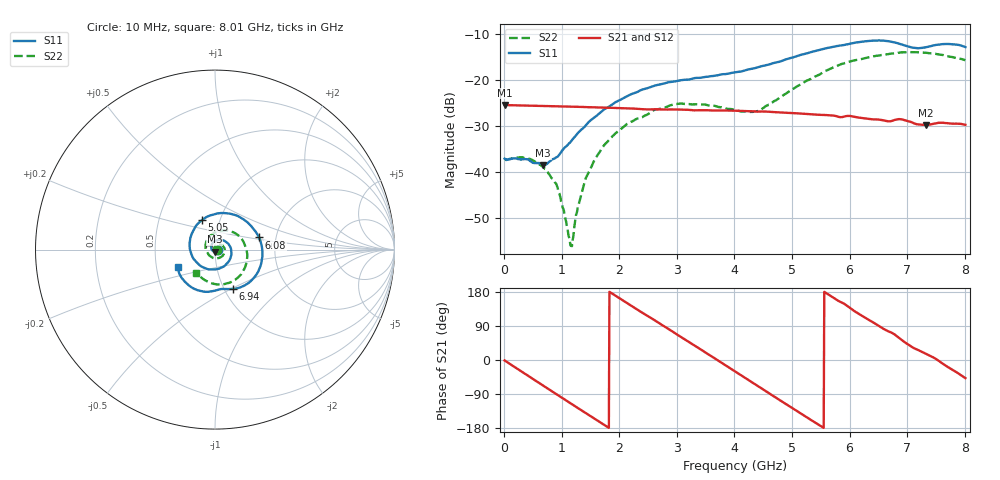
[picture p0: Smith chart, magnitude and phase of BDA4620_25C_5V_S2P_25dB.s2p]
!Agilent Technologies,E5071B,MY42404982,A.09.10
!Date: Wed May 06 09:03:50 2026
!Data & Calibration Information:
!Freq	S11:SOLT2(ON)	S21:SOLT2(ON)	S12:SOLT2(ON)	S22:SOLT2(ON)
# Hz S RI R 50
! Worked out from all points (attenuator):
!   801 points, 10 MHz to 8.01 GHz, reference 50 ohm
!   highest |S21| = -25.39 dB at 10 MHz (marker M1); lowest = -29.7 dB at 7.33 GHz (marker M2)
!   lowest |S11| = -38.5 dB at 680 MHz (marker M3), VSWR 1.02, Z = 49.8 - j1.16 ohm
!   |S11| at or under -10 dB: start of sweep to end of sweep
!   |S22| runs from -56.1 to -13.9 dB; largest |S21 - S12| = 0.00026
!   S11 on the Smith chart (normalised r, x): 10 MHz: 1.03, -0.00; 5.05 GHz: 0.82, +0.28; 6.08 GHz: 1.63, +0.24; 6.94 GHz: 1.09, -0.51; 8.01 GHz: 0.64, -0.13
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1e7  0.014 -0.000933  0.0538 -0.00111  0.0538 -0.00113  0.0135 -0.000458
4.2e8  0.00827 -0.0109  0.0394 -0.0354  0.0395 -0.0355  0.0132 -0.00462
6.8e8  -0.00218 -0.0117  0.02 -0.0486  0.02 -0.0487  0.00917 -0.00659
9.3e8  -0.0137 -0.00542  -0.00201 -0.0521  -0.00205 -0.0522  0.00349 -0.00588
1.16e9  -0.0202 0.00753  -0.0216 -0.0468  -0.0217 -0.0469  -0.00137 -0.000793
1.19e9  -0.0207 0.00964  -0.024 -0.0456  -0.024 -0.0457  -0.00181 0.000112
1.35e9  -0.0204 0.0211  -0.0352 -0.0372  -0.0352 -0.0373  -0.00332 0.00496
1.53e9  -0.0146 0.0348  -0.0444 -0.0247  -0.0444 -0.0248  -0.00307 0.0115
1.77e9  0.00199 0.0493  -0.05 -0.00514  -0.0501 -0.0051  0.00102 0.0207
2.14e9  0.0413 0.053  -0.0427 0.0248  -0.0428 0.0249  0.0169 0.0291
2.68e9  0.0891 0.00418  -0.00706 0.0476  -0.00703 0.0477  0.0445 0.0192
3.08e9  0.0812 -0.0587  0.024 0.0415  0.0242 0.0414  0.0551 -0.00764
4.01e9  -0.0835 -0.0886  0.0403 -0.0233  0.0404 -0.0234  -0.0108 -0.0465
4.43e9  -0.1396 0.00125  0.0151 -0.043  0.0151 -0.0431  -0.0451 -0.0114
5.05e9  -0.0729 0.164  -0.0288 -0.033  -0.0289 -0.033  -0.0253 0.0787
5.35e9  0.0212 0.2024  -0.04 -0.0144  -0.0401 -0.0144  0.0232 0.1022
6.08e9  0.2451 0.0679  -0.0254 0.0309  -0.0255 0.031  0.1577 0.0456
6.68e9  0.1933 -0.1811  0.00909 0.0345  0.0092 0.0346  0.1698 -0.09
6.94e9  0.098 -0.2196  0.0244 0.0278  0.0245 0.0278  0.1371 -0.1468
7.33e9  0.00168 -0.2279  0.0314 0.00912  0.0314 0.00921  0.0462 -0.193
7.65e9  -0.1156 -0.2187  0.0334 -0.00775  0.0335 -0.00776  -0.0329 -0.1826
8.01e9  -0.2084 -0.0951  0.0219 -0.0243  0.022 -0.0244  -0.1031 -0.1285
